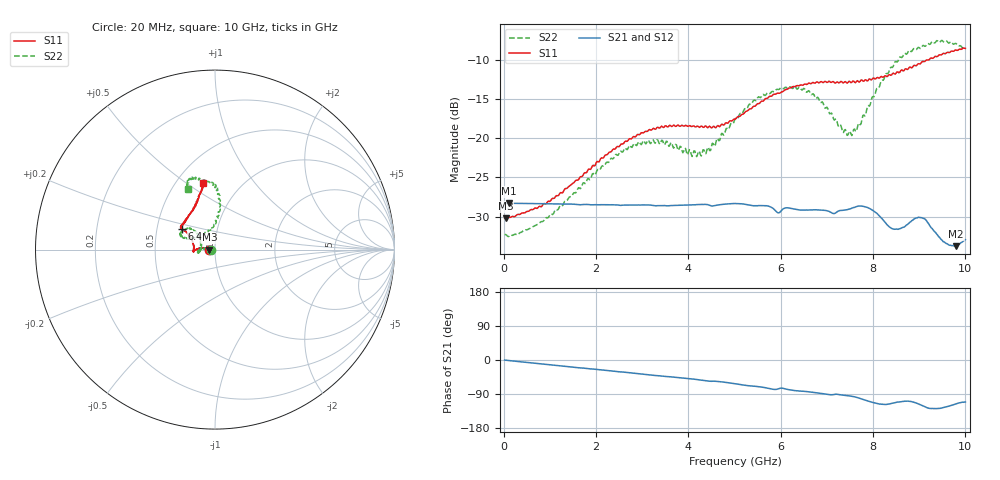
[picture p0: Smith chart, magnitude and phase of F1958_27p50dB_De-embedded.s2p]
! Integrated Device Technology
! Corporate Headquarters
! 6024 Silver Creek Valley Road
! San Jose, CA 95138  USA
! Phone:  1-408-284-8200
! Toll Free:  1-800-223-1366
! Webpage:  http://www.idt.com/
! Timing and RF Division
! 515 Groton Road, Suite 102
! Westford, MA 01886-6024
! Device:  F1958
! Description: 7-bit 0.25 dB Digital Step Attenuator
! Frequency:  0.001 -  6.000 GHz
! Package:  4x4 mm Thin QFN Plastic Package: 24 pin
! Ports:  2 RF, 12 DC
!  Pin  1  = D0
!  Pin  2  = VDD
!  Pin  3  = VMODE
!  Pin  4  = GND
!  Pin  5  = RF1  =  Port 1
!  Pin  6  = GND
!  Pin  7  = GND
!  Pin  8  = GND
!  Pin  9  = GND
!  Pin 10  = GND
!  Pin 11  = GND
!  Pin 12  = GND
!  Pin 13  = GND
!  Pin 14  = RF2  =  Port 2
!  Pin 15  = GND
!  Pin 16  = LE
!  Pin 17  = CLK
!  Pin 18  = DATA
!  Pin 19  = D6
!  Pin 20  = D5
!  Pin 21  = D4
!  Pin 22  = D3
!  Pin 23  = D2
!  Pin 24  = D1
! State:  110
! Atten State:  27.50 dB
! Voltage:  +3.30 Volts
! Current:  0.258 mA
! Data:  The device was measured on a F1958 evaluation board which has
!  individual transmission lines to the RF pins.  Data was collected
!  using a calibrated network analyzer.  The evaluation board was
!  de-embedded using Automatic Fixture Removal (AFR).
!  The reference plane is the edge of the package pin.
! Misc:
!  Action Tracker AT0419
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# GHz S dB R 50
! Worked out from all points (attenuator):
!   500 points, 20 MHz to 10 GHz, reference 50 ohm
!   highest |S21| = -28.28 dB at 120 MHz (marker M1); lowest = -33.8 dB at 9.8 GHz (marker M2)
!   lowest |S11| = -30.2 dB at 40 MHz (marker M3), VSWR 1.06, Z = 47 - j0.0429 ohm
!   |S11| at or under -10 dB: start of sweep to 9.152 GHz
!   |S22| runs from -32.6 to -7.5 dB; largest |S21 - S12| = 0.00033
!   S11 on the Smith chart (normalised r, x): 20 MHz: 0.94, -0.00; 6.4 GHz: 0.67, +0.16; 10 GHz: 0.67, +0.58
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0.02  -30.19 -178.9  -28.31 -0.2  -28.31 -0.2  -32.32 -178.8
0.04  -30.21 -179.2  -28.30 -0.4  -28.30 -0.4  -32.29 -178.3
0.12  -30.09 178.9  -28.28 -1.6  -28.29 -1.6  -32.51 178.8
0.84  -28.57 170.8  -28.35 -10.6  -28.34 -10.6  -30.64 172.4
1.7  -24.87 170.8  -28.46 -21.0  -28.46 -21.0  -25.96 171.5
2.62  -20.44 176.9  -28.53 -32.2  -28.51 -32.3  -21.26 -179.3
3.36  -18.67 -175.7  -28.60 -41.6  -28.60 -41.7  -20.53 -169.1
4.24  -18.60 -179.0  -28.46 -52.2  -28.48 -52.3  -21.67 169.1
5.02  -17.53 160.7  -28.32 -62.8  -28.34 -62.8  -17.43 138.2
5.58  -15.25 150.5  -28.59 -71.4  -28.61 -71.4  -14.68 139.9
5.94  -14.21 148.3  -29.52 -76.4  -29.54 -76.4  -13.74 148.7
6.4  -13.27 147.9  -29.15 -81.8  -29.16 -81.8  -13.44 155.9
6.68  -12.91 146.8  -29.14 -84.9  -29.15 -84.9  -14.37 158.0
7.5  -12.75 138.5  -29.02 -95.0  -29.02 -94.8  -19.09 120.3
7.68  -12.71 135.6  -28.67 -99.9  -28.67 -99.9  -18.13 99.7
7.9  -12.52 129.1  -28.89 -108.5  -28.87 -108.6  -15.80 89.2
8.34  -11.88 119.1  -31.24 -116.4  -31.25 -116.4  -11.54 83.8
8.66  -11.38 113.4  -31.35 -109.3  -31.39 -109.5  -9.30 87.6
9.06  -10.21 106.9  -30.14 -119.9  -30.20 -119.9  -8.28 97.5
9.52  -9.13 101.9  -33.22 -125.6  -33.18 -125.7  -7.63 109.3
9.8  -8.70 100.9  -33.78 -115.7  -33.74 -115.5  -7.88 112.8
10  -8.50 100.1  -32.94 -111.0  -32.99 -110.6  -8.62 114.0
